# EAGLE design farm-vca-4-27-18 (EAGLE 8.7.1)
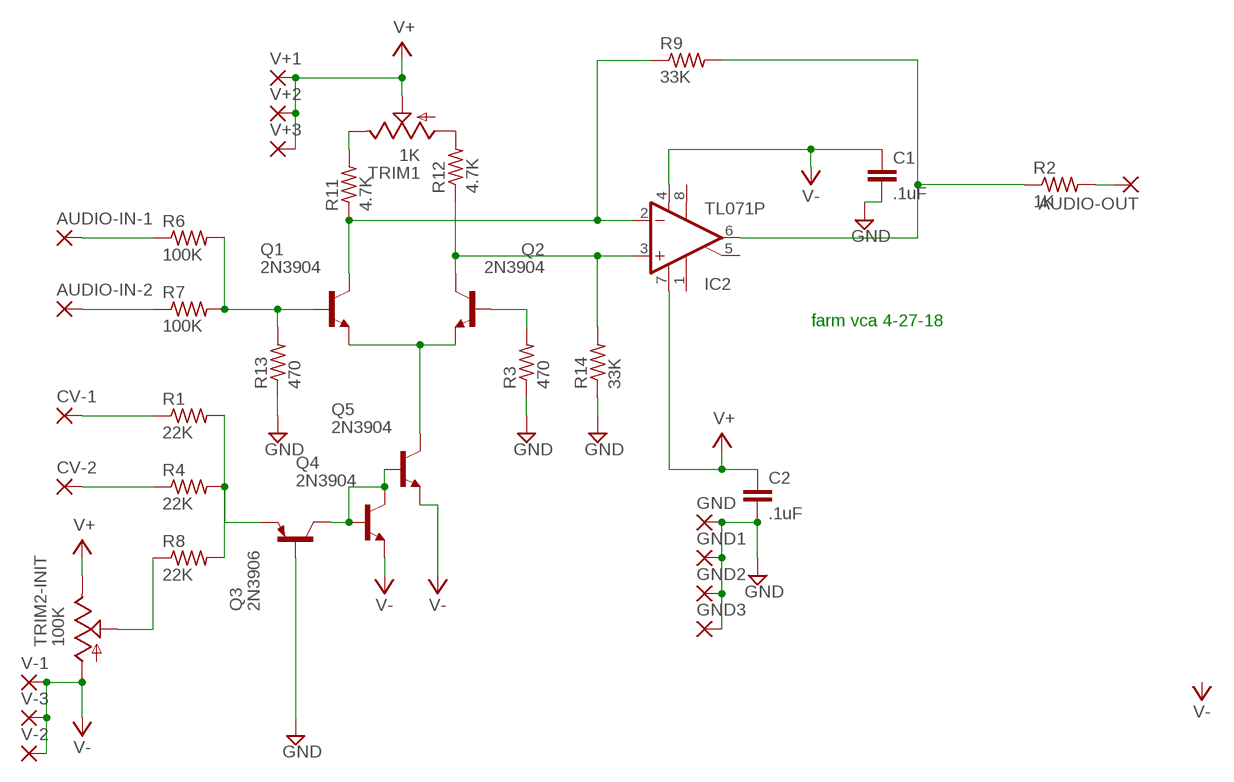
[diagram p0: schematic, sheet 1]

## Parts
AUDIO-IN-1  3,17/1,3  [3,17/1,3]
AUDIO-IN-2  3,17/1,3  [3,17/1,3]
AUDIO-OUT  3,17/1,3  [3,17/1,3]
C1  .1uF  C5/2.5  [C5B2.5]
C2  .1uF  C5/2.5  [C5B2.5]
CV-1  3,17/1,3  [3,17/1,3]
CV-2  3,17/1,3  [3,17/1,3]
GND  3,17/1,3  [3,17/1,3]
GND1  3,17/1,3  [3,17/1,3]
GND2  3,17/1,3  [3,17/1,3]
GND3  3,17/1,3  [3,17/1,3]
IC2  TL071P  [DIL08]
Q1  2N3904  [TO92]
Q2  2N3904  [TO92]
Q3  2N3906  [TO92]
Q4  2N3904  [TO92]
Q5  2N3904  [TO92]
R1  22K  R-US_0204/7  [0204/7]
R2  1K  R-US_0204/7  [0204/7]
R3  470  R-US_0204/7  [0204/7]
R4  22K  R-US_0204/7  [0204/7]
R6  100K  R-US_0204/7  [0204/7]
R7  100K  R-US_0204/7  [0204/7]
R8  22K  R-US_0204/7  [0204/7]
R9  33K  R-US_0204/7  [0204/7]
R11  4.7K  R-US_0204/7  [0204/7]
R12  4.7K  R-US_0204/7  [0204/7]
R13  470  R-US_0204/7  [0204/7]
R14  33K  R-US_0204/7  [0204/7]
TRIM1  1K  TRIM_US-S63X  [S63X]
TRIM2-INIT  100K  TRIM_US-S63X  [S63X]
V+1  3,17/1,3  [3,17/1,3]
V+2  3,17/1,3  [3,17/1,3]
V+3  3,17/1,3  [3,17/1,3]
V-1  3,17/1,3  [3,17/1,3]
V-2  3,17/1,3  [3,17/1,3]
V-3  3,17/1,3  [3,17/1,3]

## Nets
GND: C1.2 C2.2 GND1.1(P) GND2.1(P) GND3.1(P) GND.1(P) Q3.2(B) R3.1 R13.1 R14.1
N$1: R8.1 TRIM2-INIT.S
N$2: Q3.3(E) R1.2 R4.2 R8.2
N$3: CV-2.1(P) R4.1
N$4: CV-1.1(P) R1.1
N$5: Q3.1(C) Q4.1(C) Q4.2(B) Q5.2(B)
N$6: Q1.3(E) Q2.3(E) Q5.1(C)
N$8: R11.2 TRIM1.E
N$9: R12.2 TRIM1.A
N$10: IC2.2(-IN) Q1.1(C) R9.1 R11.1
N$11: IC2.3(+IN) Q2.1(C) R12.1 R14.2
N$12: Q2.2(B) R3.2
N$13: AUDIO-IN-1.1(P) R6.1
N$14: AUDIO-IN-2.1(P) R7.1
N$15: IC2.6(OUT) R2.1 R9.2
N$16: AUDIO-OUT.1(P) R2.2
N$17: Q1.2(B) R6.2 R7.2 R13.2
V+: C2.1 IC2.7(V+) TRIM1.S TRIM2-INIT.E V+1.1(P) V+2.1(P) V+3.1(P)
V-: C1.1 IC2.4(V-) Q4.3(E) Q5.3(E) TRIM2-INIT.A V-1.1(P) V-2.1(P) V-3.1(P)
Unconnected: IC2.1(ON1) IC2.5(ON2) IC2.8(OPT)

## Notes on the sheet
- farm vca 4-27-18

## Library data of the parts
AUDIO-IN-1 AUDIO-IN-2 AUDIO-OUT CV-1 CV-2 GND GND1-GND3 V+1-V+3 V-1-V-3 = wirepad:3,17/1,3: THROUGH-HOLE PAD
C1 C2 = capacitor-wima:C: CAPACITOR
IC2 = linear:TL071: OP AMP
Q1 Q2 Q4 Q5 = transistor:2N3904: NPN TRANSISTOR
Q3 = transistor-pnp:2N3906: PNP Transistor
R1-R4 R6-R9 R11-R14 = rcl:R-US_: RESISTOR, American symbol
TRIM1 TRIM2-INIT = pot:TRIM_US-: POTENTIOMETER

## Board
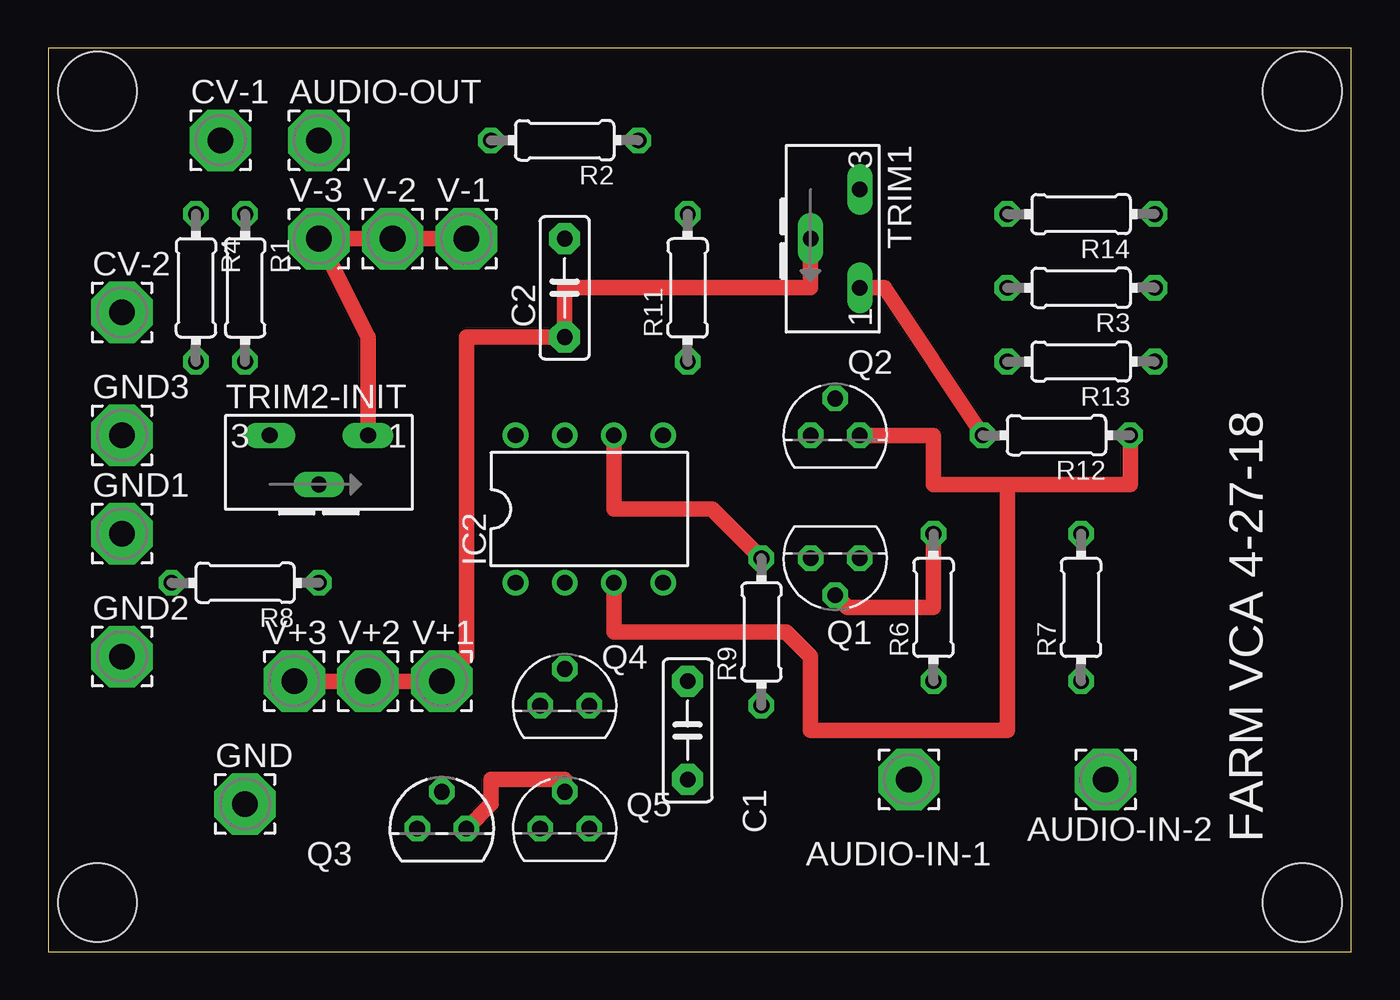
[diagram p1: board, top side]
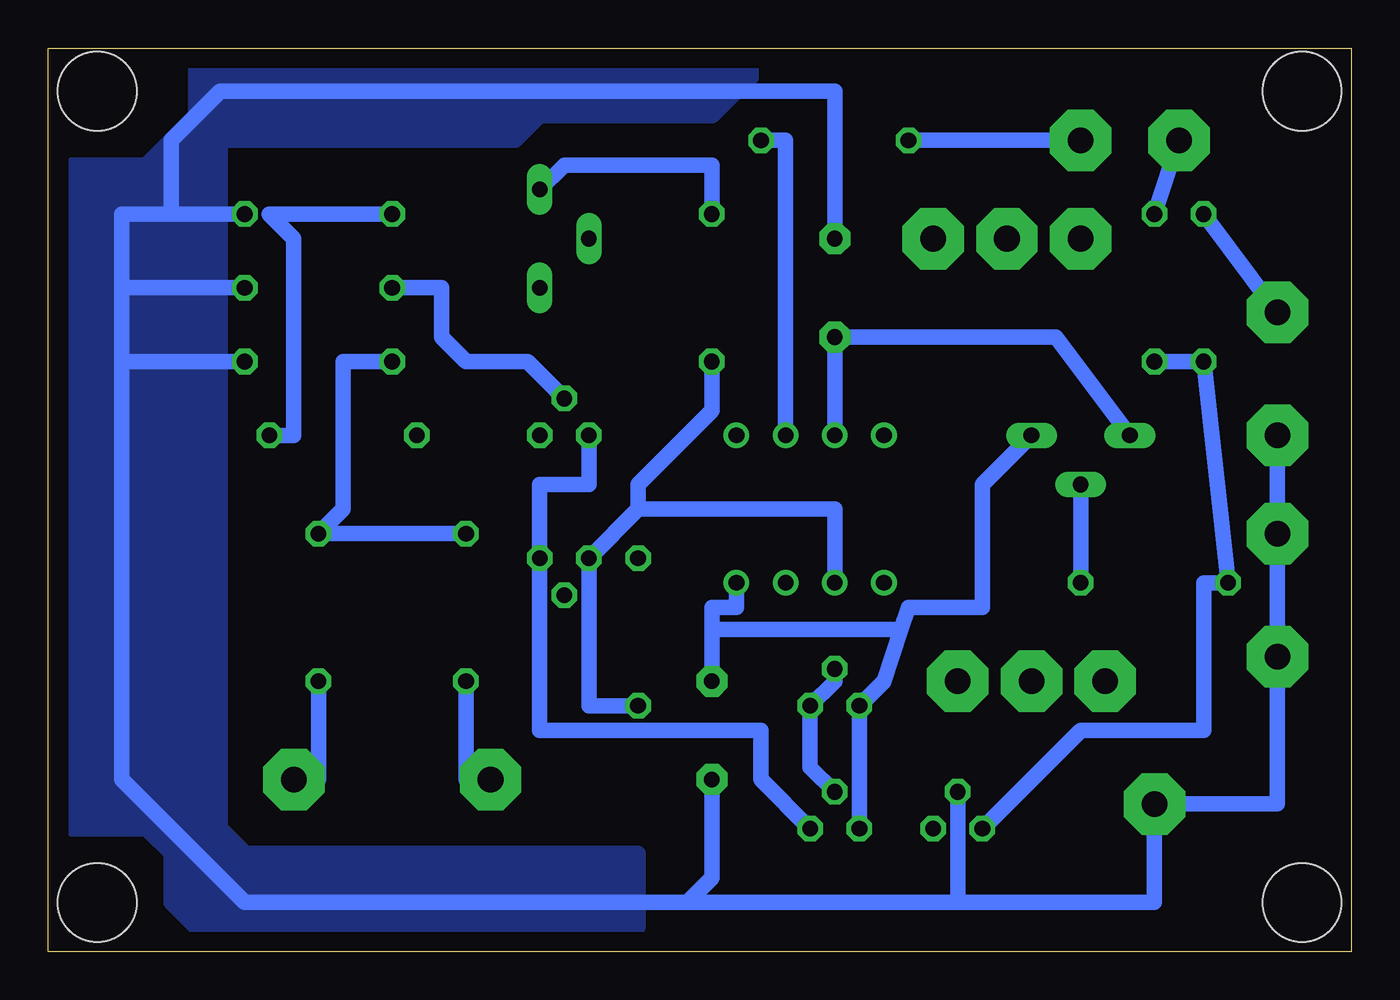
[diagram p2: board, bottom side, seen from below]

Size 67.29 x 46.66 mm. Coordinates in mm from the lower left corner, seen from the top.
Outline: 0,0 67.29,0 67.29,46.66 0,46.66 0,0
Copper layers (1*16): Top 0.035mm / dielectric 1.5mm / Bottom 0.035mm
Design rules "default": minimum track width 6mil, minimum drill 0.35mm, track to track 6mil, track to pad 6mil, pad to pad 6mil, via to via 6mil, smd to smd 6mil, copper to edge 40mil, drill to drill 6mil, minimum pad ring 10mil, minimum via ring 8mil, stop-mask expansion 4mil, vias tented up to drill 0mil, thermal gap 10mil
Holes 4.06 mm at 2.54,2.54 64.77,2.54 64.77,44.45 2.54,44.45

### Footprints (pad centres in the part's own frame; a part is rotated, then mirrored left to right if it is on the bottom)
3,17/1,3 = drill 1.321 pad 3.175 octagon: 1 0,0
C5B2.5 = drill 0.813 pad 1.6 octagon: 1 -2.54,0; 2 2.54,0
DIL08 = drill 0.813 pad 1.27: 1 -3.81,-3.81; 2 -1.27,-3.81; 3 1.27,-3.81; 4 3.81,-3.81; 5 3.81,3.81; 6 1.27,3.81; 7 -1.27,3.81; 8 -3.81,3.81
TO92 = drill 0.813 octagon: 1 1.27,0; 2 0,1.905; 3 -1.27,0
0204/7 = drill 0.813 octagon: 1 -3.81,0; 2 3.81,0
S63X = drill 0.813 long: A 2.54,0; E -2.54,0; S 0,-2.54

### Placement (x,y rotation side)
AUDIO-IN-1  44.45,8.89 0 top
AUDIO-IN-2  54.61,8.89 0 top
AUDIO-OUT  13.97,41.91 0 top
C1  33.02,11.43 270 top
C2  26.67,34.29 90 top
CV-1  8.89,41.91 0 top
CV-2  3.81,33.02 0 top
GND  10.16,7.62 0 top
GND1  3.81,21.59 0 top
GND2  3.81,15.24 0 top
GND3  3.81,26.67 0 top
IC2  27.94,22.86 0 top
Q1  40.64,20.32 180 top
Q2  40.64,26.67 0 top
Q3  20.32,6.35 0 top
Q4  26.67,12.7 0 top
Q5  26.67,6.35 0 top
R1  10.16,34.29 270 top
R2  26.67,41.91 180 top
R3  53.34,34.29 180 top
R4  7.62,34.29 270 top
R6  45.72,17.78 90 top
R7  53.34,17.78 90 top
R8  10.16,19.05 180 top
R9  36.83,16.51 90 top
R11  33.02,34.29 90 top
R12  52.07,26.67 180 top
R13  53.34,30.48 180 top
R14  53.34,38.1 180 top
TRIM1  41.91,36.83 270 top
TRIM2-INIT  13.97,26.67 0 top
V+1  20.32,13.97 0 top
V+2  16.51,13.97 0 top
V+3  12.7,13.97 0 top
V-1  21.59,36.83 0 top
V-2  17.78,36.83 0 top
V-3  13.97,36.83 0 top

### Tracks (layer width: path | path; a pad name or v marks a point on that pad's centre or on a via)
GND
  Bottom 0.813: 20.32,2.54 34.29,2.54 | 34.29,2.54 33.02,3.81 C1.2 | 34.29,2.54 57.15,2.54 63.5,8.89 63.5,30.48 | 63.5,30.48 63.5,34.29 | 63.5,34.29 63.5,38.1 60.96,38.1 | C2.2 26.67,44.45 58.42,44.45 60.96,41.91 60.96,38.1 | R3.1 63.5,34.29 | R14.1 60.96,38.1 | R13.1 63.5,30.48 | Q3.2 20.32,2.54 | GND3.1 GND1.1 GND2.1 3.81,7.62 GND.1 10.16,2.54 20.32,2.54
  pour Bottom: 36.83,5.08 36.83,1.27 59.69,1.27 60.96,2.54 60.96,5.08 62.23,6.35 66.04,6.35 66.04,40.64 62.23,40.64 59.69,43.18 59.69,45.72 30.48,45.72 33.02,43.18 41.91,43.18 43.18,41.91 58.42,41.91 58.42,7.62 58.42,6.35 57.15,5.08
N$1
  Bottom 0.813: R8.1 TRIM2-INIT.S
N$2
  Bottom 0.813: R1.2 R4.2 R8.2 7.62,19.05 7.62,11.43 13.97,11.43 Q3.3
N$3
  Bottom 0.813: CV-2.1 R4.1
N$4
  Bottom 0.813: CV-1.1 R1.1
N$5
  Top 0.813: Q3.1 22.86,7.62 22.86,8.89 26.67,8.89 Q5.2
  Bottom 0.813: Q5.2 27.94,9.53 Q4.1 26.67,13.97 Q4.2
N$6
  Bottom 0.813: Q5.1 30.48,8.89 30.48,11.43 41.91,11.43 Q1.3 41.91,24.13 39.37,24.13 Q2.3
N$8
  Bottom 0.813: R11.2 33.02,40.64 40.64,40.64 TRIM1.E
N$9
  Top 0.813: TRIM1.A 43.18,34.29 R12.2
N$10
  Bottom 0.813: R11.1 33.02,27.94 36.83,24.13 36.83,22.86 | 36.83,22.86 Q1.1 39.37,12.7 R9.1 | IC2.2 26.67,22.86 36.83,22.86
N$11
  Top 0.813: IC2.3 29.21,16.51 38.1,16.51 39.37,15.24 39.37,11.43 49.53,11.43 49.53,24.13 | 49.53,24.13 55.88,24.13 R12.1 | Q2.1 45.72,26.67 45.72,24.13 49.53,24.13
  Bottom 0.813: R12.1 54.61,26.67 54.61,36.83 55.88,38.1 R14.2
N$12
  Bottom 0.813: Q2.2 42.55,30.48 45.72,30.48 46.99,31.75 46.99,34.29 R3.2
N$13
  Bottom 0.813: AUDIO-IN-1.1 45.72,8.89 R6.1
N$14
  Bottom 0.813: R7.1 53.34,8.89 AUDIO-IN-2.1
N$15
  Top 0.813: R9.2 34.29,22.86 29.21,22.86 IC2.6
  Bottom 0.813: IC2.6 29.21,41.91 R2.1
N$16
  Bottom 0.813: R2.2 AUDIO-OUT.1
N$17
  Top 0.813: Q1.2 41.28,17.78 45.72,17.78 R6.2
  Bottom 0.813: R6.2 R7.2 52.07,22.86 52.07,30.48 R13.2
V+
  Top 0.813: TRIM1.S 39.37,34.29 26.67,34.29 C2.1 21.59,31.75 21.59,15.24 V+1.1 V+2.1 V+3.1
  Bottom 0.813: IC2.7 C2.1 15.24,31.75 TRIM2-INIT.E
V-
  Top 0.813: TRIM2-INIT.A 16.51,31.75 V-3.1 V-2.1 V-1.1
  Bottom 0.813: 23.24,16.64 24.13,13.97 Q4.3 Q5.3 | 23.24,16.64 22.86,17.78 19.05,17.78 19.05,24.13 TRIM2-INIT.A | C1.1 33.02,16.51 | 33.02,16.51 33.02,17.78 31.75,17.78 IC2.4 | 33.02,16.51 32.89,16.64 23.24,16.64

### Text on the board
tNames: FARM VCA 4-27-18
